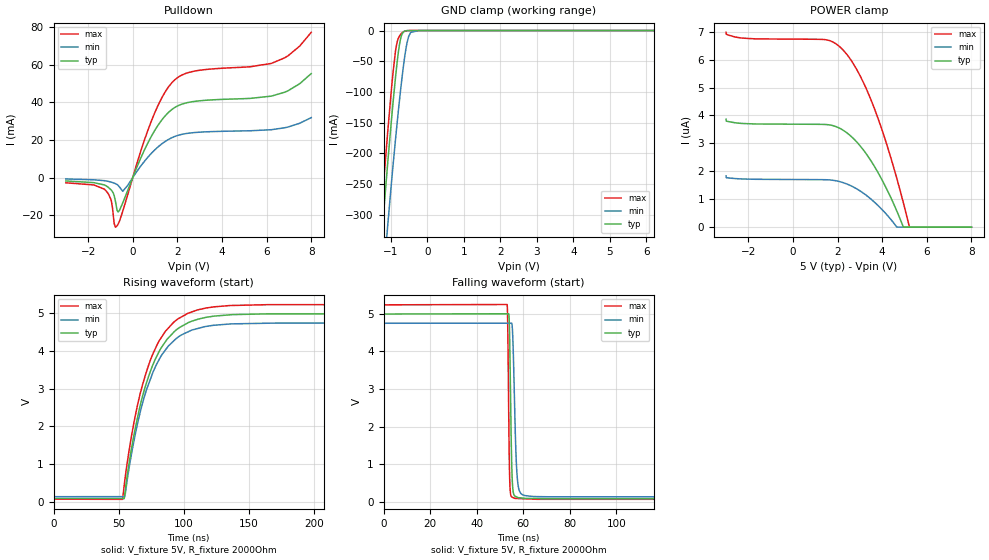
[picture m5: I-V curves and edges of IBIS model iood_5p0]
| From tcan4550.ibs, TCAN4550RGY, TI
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|   iood_5p0 Model
[Model]   iood_5p0
Model_type   I/O_open_drain
Polarity   Inverting
Enable   Active-High
Vinl = 1.5
Vinh = 3.5
Vmeas = 2.5
Vref = 5
Cref = 2pF
Rref = 2000
|   typ   min   max
C_comp   5.031pF   4.760pF   5.172pF
|  Where Nom  PVT is Nominal Process, 5V,   27C
|   Fast PVT is Strong Process,  5.25, -40C
|   Slow PVT is Weak Process,   4.75V, 150C
[Model spec]
|subparameter
Vinl   1.5   1.425   1.575
Vinh   3.5   3.325   3.675
[Voltage Range]   5   4.75   5.25
|Junction Temperature
[Temperature Range]   27   150   -40
[Pullup Reference]   5   4.75   5.25
[Pulldown Reference]   0   -0   0
[Power Clamp Reference]   5   4.75   5.25
[GND Clamp Reference]   0   0   0
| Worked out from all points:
|   slope of the pulldown table from 0 to 0.75 V, typ, clamps not added: 37.4 ohm
|   GND clamp passes 1 mA (typ) near -0.62 V on its own axis
|   falling waveform, V_fixture 5V, R_fixture 2000Ohm: 20-80 % time 766ps typ, 1.23ns min, 569ps max; typ from 4.99 V to 0.081 V
|   rising waveform, V_fixture 5V, R_fixture 2000Ohm: 20-80 % time 23.2ns typ, 23ns min, 23.1ns max; typ from 0.081 V to 4.99 V
[Pulldown]
|   Voltage   I(typ)   I(min)   I(max)
-3V       -1.784mA   -714.8uA   -2.754mA
-1.273V   -3.897mA   -1.629mA   -6.114mA
-976mV    -6.443mA   -2.366mA   -11.6mA
-767mV    -13.13mA   -3.25mA    -26.32mA
-591mV    -17.36mA   -5.026mA   -23.04mA
-448mV    -13.45mA   -7.26mA    -17.87mA
839mV     22.01mA    12.93mA    30.13mA
1.818V    36.71mA    21.53mA    51.17mA
2.841V    40.58mA    23.99mA    56.71mA
6.218V    43.28mA    25.44mA    60.65mA
6.966V    46.16mA    26.89mA    64.75mA
8V        55.25mA    31.86mA    77.16mA
[GND Clamp]
|   Voltage   I(typ)   I(min)   I(max)
-3V       -1.78A     -1.815A    -1.774A
-1.526V   -551.6mA   -641.1mA   -509mA
-1.273V   -351.5mA   -450mA     -303.3mA
-1.218V   -309.7mA   -409.6mA   -260.6mA
-1.086V   -213.4mA   -315.5mA   -163.1mA
-877mV    -77.54mA   -178.4mA   -34.22mA
-745mV    -15.9mA    -101.9mA   -7.128mA
-624mV    -1.034mA   -43mA      -1.096mA
-558mV    -207.8uA   -19.64mA   -238.1uA
-459mV    -16.22uA   -3.106mA   -14.57uA
-239mV    -395.8nA   -11.2uA    -697.7nA
8V        0A         0A         0A
[POWER Clamp]
|   Voltage   I(typ)   I(min)   I(max)
-3V       3.864uA    1.836uA    6.976uA
-2.263V   3.712uA    1.725uA    6.768uA
1.455V    3.676uA    1.698uA    6.712uA
2.016V    3.57uA     1.645uA    6.512uA
2.423V    3.373uA    1.543uA    6.176uA
2.841V    3.065uA    1.379uA    5.668uA
3.556V    2.298uA    962.8nA    4.438uA
4.073V    1.566uA    561.8nA    3.283uA
4.645V    592.7nA    9.881nA    1.772uA
4.942V    13.2nA     0A         886.8nA
5.217V    0A         0A         8.036nA
8V        0A         0A         0A
[Ramp]
R_load = 2000
|   typ   min   max
dV/dt_r   2.94681/2.32078e-08   2.77006/2.30489e-08   3.10372/2.31589e-08
dV/dt_f   2.94681/7.63042e-10   2.77006/1.23327e-09   3.10372/5.67949e-10
[Falling Waveform]
V_fixture = 5V
V_fixture_min = 4.75V
V_fixture_max = 5.25V
R_fixture = 2000Ohm
C_fixture = 0F
|   Time   V(typ)   V(min)   V(max)
0s        4.992V     4.746V     5.236V
53.03ns   4.999V     4.748V     5.245V
53.35ns   4.999V     4.748V     4.501V
53.92ns   4.866V     4.748V     1.353V
54.52ns   2.845V     4.748V     209.8mV
55.34ns   468.6mV    4.567V     116.2mV
56.74ns   138.9mV    1.475V     87.74mV
57.7ns    109.8mV    465.4mV    85.27mV
65.82ns   83.75mV    136.2mV    64.34mV
25us      81.14mV    129.7mV    63.54mV
[Rising Waveform]
V_fixture = 5V
V_fixture_min = 4.75V
V_fixture_max = 5.25V
R_fixture = 2000Ohm
C_fixture = 0F
|   Time   V(typ)   V(min)   V(max)
0s        81.14mV    129.7mV    63.54mV
52.93ns   79.51mV    131.2mV    59.61mV
54.91ns   258.2mV    172.7mV    623.9mV
59.68ns   1.379V     1.237V     1.712V
68.02ns   2.766V     2.58V      3.072V
78.88ns   3.839V     3.636V     4.123V
92.02ns   4.492V     4.263V     4.759V
117ns     4.895V     4.654V     5.142V
164.9ns   4.988V     4.739V     5.232V
25us      4.992V     4.746V     5.236V
